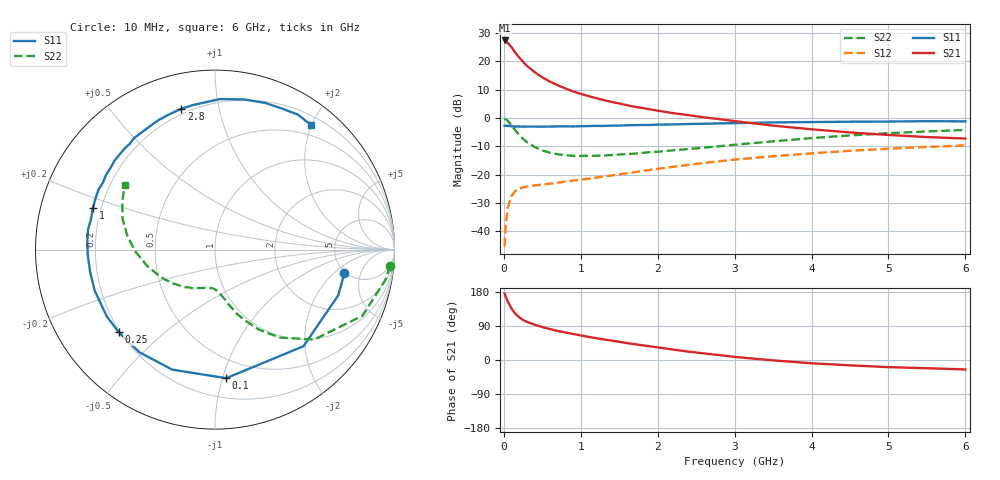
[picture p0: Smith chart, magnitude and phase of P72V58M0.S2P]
! SIEMENS Small Signal Semiconductors
! BFP196
! Si NPN RF Bipolar Junction Transistor in SOT143
! VCE = 2.5 V  IC = 8 mA
! Common Emitter S-Parameters:  May  1996
# GHz  S  MA  R  50
!  f  S11  S21  S12  S22
! GHz  MAG  ANG  MAG  ANG  MAG  ANG  MAG  ANG
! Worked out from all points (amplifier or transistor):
!   36 points, 10 MHz to 6 GHz, reference 50 ohm
!   highest |S21| = 27.4 dB at 10 MHz (marker M1)
!   |S21| within 3 dB of that: start of sweep to 115.7 MHz
!   unconditionally stable (mu >= 1): 932.8 MHz to 3.327 GHz
!   at 250 MHz: K = 0.35, MSG = 22.1 dB, |S12| = -24.4 dB
!   at 1.4 GHz: K = 1.15, MAG = 10.6 dB, |S12| = -20.3 dB
!   at 6 GHz: K = 0.99, MSG = 1.2 dB, |S12| = -9.6 dB
!   S11 on the Smith chart (normalised r, x): 10 MHz: 4.84, -2.76; 100 MHz: 0.35, -1.03; 250 MHz: 0.19, -0.36; 1 GHz: 0.17, +0.16; 2.8 GHz: 0.17, +0.78; 6 GHz: 0.33, +1.98
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0.01  0.7323 -10.4  23.45 175.5  0.0055 86.4  0.9801 -5.3
0.02  0.7327 -20.3  22.92 169.1  0.0109 80.9  0.9642 -10.1
0.05  0.73 -47.5  21.38 154.9  0.0257 67.0  0.9006 -24.1
0.1  0.7191 -85.0  17.82 135.6  0.0426 52.3  0.7463 -42.2
0.15  0.71 -109.6  14.23 121.9  0.0519 42.0  0.6068 -53.8
0.2  0.7106 -126.5  11.75 112.8  0.0571 36.5  0.5061 -61.4
0.25  0.7065 -139.5  9.784 105.7  0.06 32.9  0.4298 -66.9
0.3  0.7086 -148.3  8.382 100.7  0.062 31.3  0.3785 -71.1
0.4  0.7082 -161.2  6.478 93.2  0.0648 29.1  0.3093 -76.5
0.5  0.7069 -170.0  5.231 86.9  0.0675 29.4  0.2691 -80.4
0.6  0.7097 -177.7  4.405 81.6  0.0697 30.2  0.2446 -84.0
0.7  0.7132 176.0  3.806 76.7  0.0724 31.5  0.2303 -87.3
0.8  0.7162 171.1  3.332 72.6  0.0758 32.5  0.2214 -90.3
1  0.719 161.0  2.68 64.8  0.0821 35.2  0.2153 -95.4
1.1  0.7238 156.9  2.447 61.1  0.0853 36.4  0.2158 -98.4
1.6  0.7476 138.6  1.688 44.7  0.1068 40.7  0.2324 -112.9
2.2  0.7735 119.9  1.224 27.6  0.1382 41.2  0.2702 -129.5
2.8  0.8069 103.4  0.959 12.9  0.1731 37.9  0.3189 -147.5
3.5  0.8393 88.1  0.737 -1.0  0.2124 31.2  0.389 -166.6
4.5  0.8637 71.1  0.559 -14.1  0.2651 20.3  0.495 170.9
5.5  0.8825 58.4  0.463 -21.7  0.3101 8.6  0.5823 152.5
6  0.8767 52.6  0.436 -24.9  0.3298 2.3  0.6179 144.3
